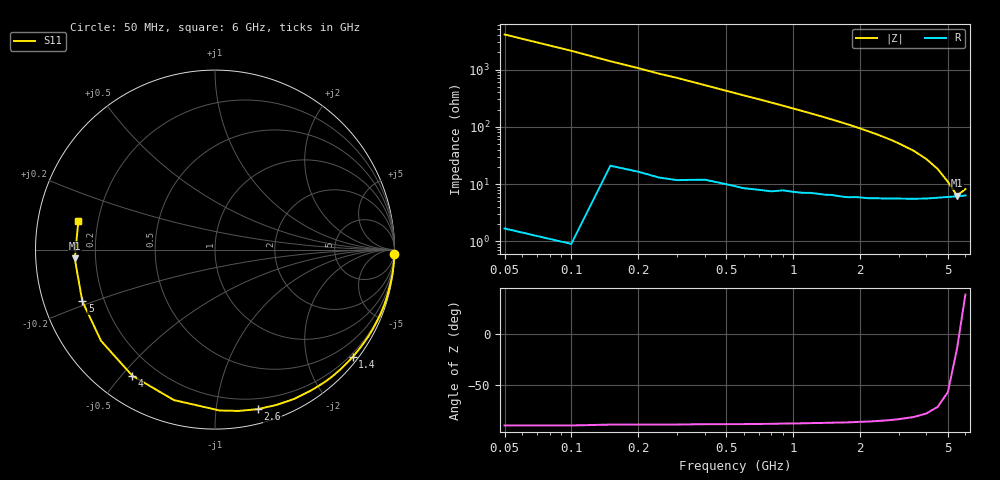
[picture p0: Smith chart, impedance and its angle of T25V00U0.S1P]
! SIEMENS Discrete & RF Semiconductors
! BAS70-04W
! Si Schottky Diode in SOT323
! VR = 5 V
! S-Parameters:  November  1997
# GHz  S  MA  R  50
!  f  S11
! GHz  MAG  ANG
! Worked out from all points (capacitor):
!   34 points, 50 MHz to 6 GHz, reference 50 ohm
!   read as one part to ground: C = 759 fF near 50 MHz
!   lowest |Z| = 6.28 ohm at 5.5 GHz (marker M1)
!   series resonance near 5.615 GHz, so ESL is about 1.1 nH
!   S11 on the Smith chart (normalised r, x): 50 MHz: 0, -82; 1.4 GHz: 0.13, -2.90; 2.6 GHz: 0.11, -1.30; 4 GHz: 0.11, -0.53; 5 GHz: 0.12, -0.18; 6 GHz: 0.13, +0.10
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0.05  1 -1.4
0.1  1 -2.7
0.25  0.9982 -6.8
0.3  0.9977 -8.0
0.4  0.9959 -10.7
0.6  0.9934 -16.1
0.7  0.9916 -18.7
0.8  0.9898 -21.4
0.9  0.9865 -24.1
1  0.9842 -26.9
1.1  0.9818 -29.6
1.3  0.9755 -35.2
1.4  0.9727 -38.0
1.6  0.9661 -43.8
1.7  0.9629 -46.8
1.8  0.9592 -49.7
2  0.9496 -55.9
2.2  0.9415 -62.1
2.4  0.9307 -68.4
2.6  0.9203 -75.0
2.8  0.9087 -81.5
3  0.897 -88.3
3.5  0.8691 -105.3
4  0.8401 -123.3
4.5  0.8134 -141.3
5  0.7932 -158.8
5.5  0.7831 -176.4
6  0.7778 168.0
